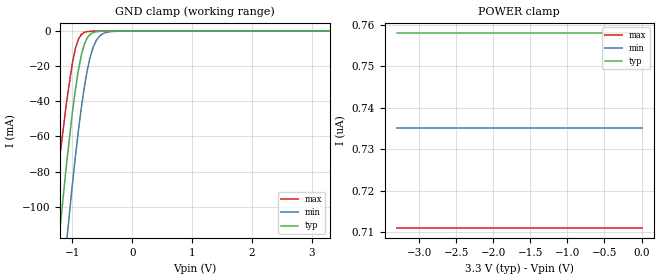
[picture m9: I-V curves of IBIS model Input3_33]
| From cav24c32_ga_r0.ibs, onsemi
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|//////////////////////////////////////////////////////////////////////////////
|//////////////////////////////////////////////////////////////////////////////
[Model]  Input3_33
Model_type Input
Vinh = 2.31
Vinl = 0.99
|  variable   typ   min   max
C_comp   6pF   6pF   6pF
|//////////////////////////////////////////////////////////////////////////////
[Temperature Range]   25   125   -40
|//////////////////////////////////////////////////////////////////////////////
[Voltage Range]   3.30V   3.00V   3.60V
|//////////////////////////////////////////////////////////////////////////////
[POWER Clamp Reference] 3.30V   3.00V   3.60V
|//////////////////////////////////////////////////////////////////////////////
[GND Clamp Reference]   0V   0V   0V
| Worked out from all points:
|   GND clamp passes 1 mA (typ) near -0.66 V on its own axis
|//////////////////////////////////////////////////////////////////////////////
[GND Clamp]
|   Voltage   I(typ)   I(min)   I(max)
-3.3V     -949mA     -1.05A     -799mA
-1.4V     -182mA     -235mA     -131mA
-1.3V     -145mA     -196mA     -99.3mA
-1.2V     -110mA     -158mA     -68.8mA
-1.1V     -76.2mA    -121mA     -40.9mA
-950mV    -33.3mA    -71.4mA    -9.9mA
-850mV    -13.5mA    -43.4mA    -1.85mA
-800mV    -7.37mA    -31.8mA    -683uA
-650mV    -767uA     -8.91mA    -43.7uA
-550mV    -153uA     -2.96mA    -17.2uA
-400mV    -18.5uA    -474uA     -10uA
3.3V      758nA      735nA      711nA
|//////////////////////////////////////////////////////////////////////////////
[POWER Clamp]
|   Voltage   I(typ)   I(min)   I(max)
-3.3V     758nA      735nA      711nA
-3.2V     758nA      735nA      711nA
-3.1V     758nA      735nA      711nA
0V        758nA      735nA      711nA
